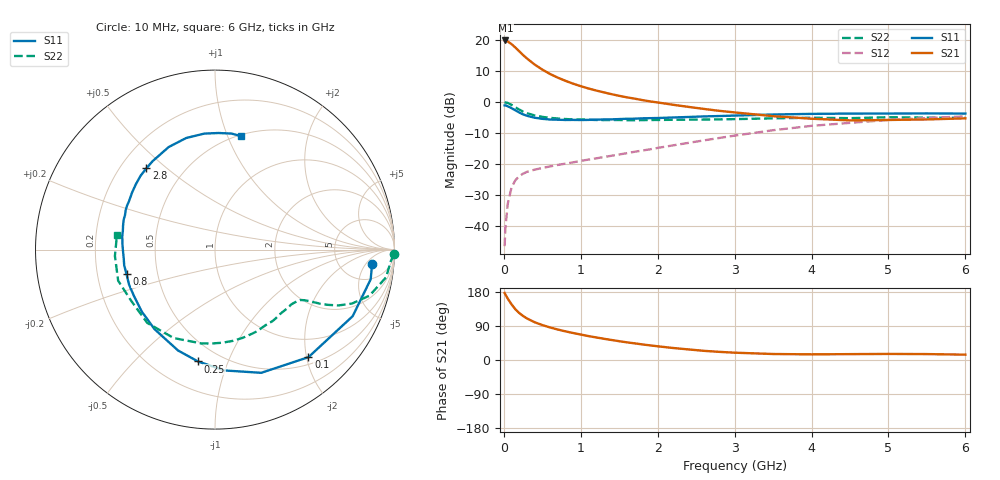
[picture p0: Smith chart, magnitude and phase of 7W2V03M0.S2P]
! Infineon Technologies  Discrete & RF Semiconductors
! BFS17W
! Si NPN RF Bipolar Junction Transistor in SOT323
! VCE = 2 V  IC = 3 mA
! Common Emitter S-Parameters:  August  1999
# GHz  S  MA  R  50
!  f  S11  S21  S12  S22
! GHz  MAG  ANG  MAG  ANG  MAG  ANG  MAG  ANG
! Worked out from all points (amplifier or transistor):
!   36 points, 10 MHz to 6 GHz, reference 50 ohm
!   highest |S21| = 19.9 dB at 20 MHz (marker M1)
!   |S21| within 3 dB of that: start of sweep to 179.4 MHz
!   unconditionally stable (mu >= 1): 682.5 MHz to end of sweep
!   at 250 MHz: K = 0.45, MSG = 19.2 dB, |S12| = -23.2 dB
!   at 1.4 GHz: K = 1.31, MAG = 6.6 dB, |S12| = -17.4 dB
!   at 6 GHz: K = 1.11, MAG = -2.3 dB, |S12| = -4.7 dB
!   S11 on the Smith chart (normalised r, x): 10 MHz: 10, -7; 100 MHz: 0.63, -2.04; 250 MHz: 0.38, -0.79; 800 MHz: 0.33, -0.12; 2.8 GHz: 0.31, +0.43; 6 GHz: 0.51, +1.12
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0.01  0.879 -5.2  9.824 177.0  0.0047 84.5  0.9967 -1.4
0.02  0.883 -10.8  9.833 172.9  0.0091 86.7  0.9815 -3.8
0.05  0.8521 -25.8  9.489 162.2  0.0224 76.2  0.9656 -9.2
0.1  0.7939 -49.0  8.588 146.9  0.0417 64.9  0.8981 -16.6
0.15  0.7334 -69.4  7.549 133.9  0.0545 55.9  0.8203 -21.5
0.2  0.6756 -85.4  6.577 124.0  0.0634 50.9  0.7535 -24.4
0.25  0.6305 -98.6  5.721 116.2  0.0695 46.4  0.6994 -26.1
0.3  0.5987 -110.1  5.04 109.7  0.0744 44.3  0.6608 -27.2
0.4  0.5568 -127.3  4.022 99.7  0.0808 41.9  0.6051 -28.5
0.5  0.5343 -139.9  3.33 92.2  0.0858 41.4  0.5746 -29.4
0.6  0.5206 -149.7  2.83 85.9  0.0911 42.0  0.5536 -30.5
0.8  0.5117 -164.4  2.196 75.6  0.101 44.8  0.5302 -34.1
0.9  0.5134 -170.2  1.973 71.3  0.1059 46.4  0.5227 -35.9
1.1  0.5133 -179.9  1.65 63.1  0.1174 49.1  0.5159 -40.6
1.3  0.5221 171.7  1.428 56.0  0.1293 51.8  0.5096 -45.9
1.6  0.5354 161.9  1.187 46.6  0.1491 55.0  0.5074 -54.2
2.2  0.5615 145.2  0.901 31.7  0.1992 59.4  0.5153 -72.6
2.8  0.5924 130.2  0.719 21.5  0.2621 59.5  0.5235 -92.1
3.5  0.627 114.3  0.59 15.8  0.3497 55.4  0.5438 -115.0
4.5  0.649 95.3  0.504 15.5  0.4597 43.8  0.5472 -148.5
5.5  0.6529 82.0  0.522 15.6  0.5501 31.8  0.5587 -176.4
6  0.6491 77.0  0.544 14.1  0.5851 26.1  0.5523 171.3
